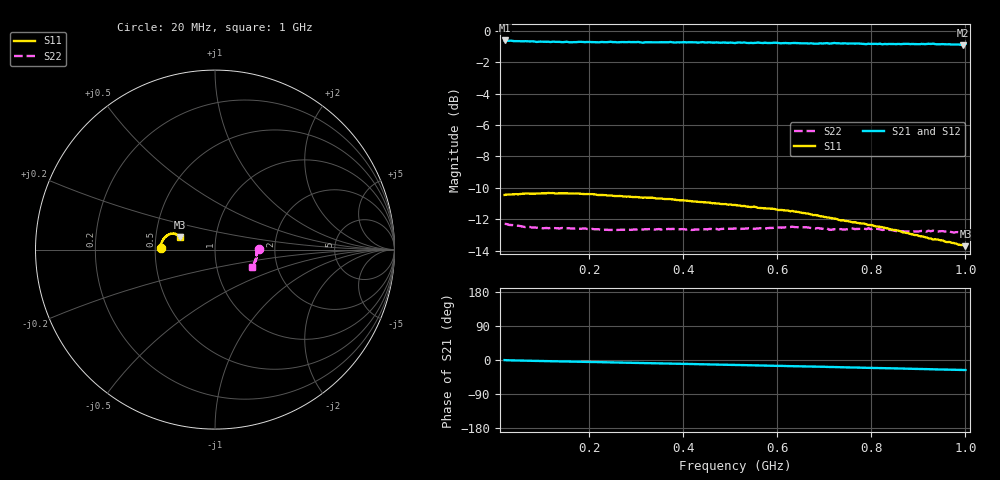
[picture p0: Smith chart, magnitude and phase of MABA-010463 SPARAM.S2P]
!Agilent Technologies,E5070B,MY42100206,A.09.10
!Date: Thu Sep 02 11:27:37 2010
!Data & Calibration Information:
!Freq	S11:SOLT2(ON)	S21:SOLT2(ON)	S12:SOLT2(ON)	S22:SOLT2(ON)
# Hz S dB R 75
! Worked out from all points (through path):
!   201 points, 20 MHz to 1 GHz, reference 75 ohm
!   highest |S21| = -0.61 dB at 20 MHz (marker M1); lowest = -0.9 dB at 995.1 MHz (marker M2)
!   group delay of S21, straight-line fit = 72.8 ps
!   lowest |S11| = -13.7 dB at 1 GHz (marker M3), VSWR 1.52, Z = 50.2 + j7.33 ohm
!   |S11| at or under -10 dB: start of sweep to end of sweep
!   |S22| runs from -12.9 to -12.3 dB; largest |S21 - S12| = 0.022
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2e7  -10.45 178.8  -0.61 -0.3  -0.62 -0.4  -12.29 0.6
3.47e7  -10.41 178.8  -0.62 -0.9  -0.63 -1.1  -12.37 -0.9
7.39e7  -10.38 177.7  -0.67 -2.2  -0.68 -2.1  -12.50 -2.4
1.866e8  -10.39 173.8  -0.70 -4.8  -0.71 -4.8  -12.60 -3.9
2.552e8  -10.53 171.3  -0.71 -6.5  -0.72 -6.3  -12.69 -5.0
3.483e8  -10.69 168.2  -0.73 -8.8  -0.71 -8.7  -12.63 -6.6
4.316e8  -10.89 165.7  -0.75 -11.0  -0.72 -10.7  -12.65 -7.8
4.414e8  -10.92 165.6  -0.71 -11.2  -0.72 -10.9  -12.66 -7.9
5.1e8  -11.09 163.7  -0.77 -13.1  -0.72 -12.5  -12.59 -9.4
5.59e8  -11.28 162.7  -0.74 -14.3  -0.73 -13.8  -12.59 -10.3
6.031e8  -11.42 161.7  -0.77 -15.6  -0.72 -15.0  -12.53 -11.2
6.08e8  -11.41 161.7  -0.79 -15.5  -0.72 -14.8  -12.54 -11.3
6.325e8  -11.47 161.1  -0.77 -16.5  -0.73 -15.6  -12.48 -11.6
6.766e8  -11.75 159.9  -0.81 -17.4  -0.71 -16.7  -12.57 -12.4
7.207e8  -11.96 159.4  -0.77 -18.6  -0.73 -17.8  -12.63 -13.6
7.942e8  -12.38 158.7  -0.81 -20.7  -0.72 -19.8  -12.58 -15.9
8.383e8  -12.63 158.6  -0.83 -21.9  -0.74 -21.0  -12.69 -17.7
8.726e8  -12.86 158.7  -0.82 -22.8  -0.76 -21.8  -12.80 -19.1
9.314e8  -13.30 158.9  -0.81 -24.5  -0.73 -23.5  -12.73 -21.3
9.363e8  -13.28 159.1  -0.85 -24.8  -0.75 -23.6  -12.77 -21.6
9.951e8  -13.66 159.6  -0.91 -26.3  -0.78 -25.1  -12.92 -24.7
1e9  -13.72 160.2  -0.84 -26.4  -0.77 -25.5  -12.85 -25.1
